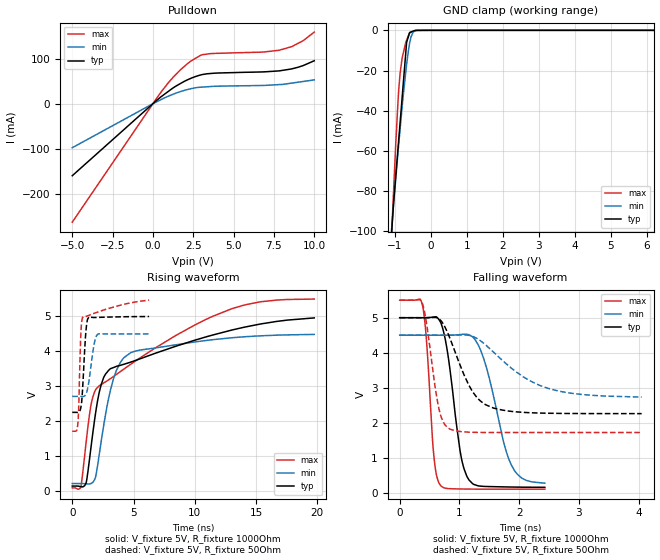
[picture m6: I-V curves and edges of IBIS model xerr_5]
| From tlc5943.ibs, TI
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|   xerr_5 Model
[Model]   xerr_5
Model_type   Open_drain
Polarity   Inverting
Vmeas = 2.5
Vref = 5.0
Cref = 15pF
Rref = 1000
|   typ   min   max
|   (nom PVT)   (Fast PVT)   (slow PVT)
C_comp   1.152e-12   1.144e-12   1.154e-12
|ON state : BUFFER OUTPUT TURNED LOW
|C_comp   2.072e-12   1.804e-12   2.153e-12
|OFF state: BUFFER IN HIGH IMPEDANCE
|C_comp   1.152e-12   1.144e-12   1.154e-12
| Where nom  PVT is Nominal Process,  5V,  65C
|   Fast PVT is Strong Process,   5.5V,  -40C
|   Slow PVT is Weak Process,   4.5V,  125C
[Voltage Range]   5   4.5   5.5
|Ambient Temperature   25   85   -40
|Junction Temperature
[Temperature Range]   65   125   -40
[Pullup Reference]   5   4.5   5.5
[Pulldown Reference]   0   0   0
[Power Clamp Reference]   5   4.5   5.5
[GND Clamp Reference]   0   0   0
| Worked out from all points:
|   slope of the pulldown table from 0 to 0.75 V, typ, clamps not added: 34.3 ohm
|   GND clamp passes 1 mA (typ) near -0.58 V on its own axis
|   falling waveform, V_fixture 5V, R_fixture 1000Ohm: 20-80 % time 220ps typ, 357ps min, 120ps max; typ from 5 V to 0.155 V
|   rising waveform, V_fixture 5V, R_fixture 1000Ohm: 20-80 % time 5.71ns typ, 1.64ns min, 7.21ns max; typ from 0.153 V to 4.96 V
|   rising waveform, V_fixture 5V, R_fixture 50Ohm: 20-80 % time 264ps typ, 426ps min, 205ps max; typ from 2.26 V to 5 V
|   falling waveform, V_fixture 5V, R_fixture 50Ohm: 20-80 % time 422ps typ, 830ps min, 190ps max; typ from 5 V to 2.26 V
[Pulldown]
|   Voltage   I(typ)   I(min)   I(max)
-5V       -159.5mA   -97.5mA    -262.4mA
561mV     16.88mA    10.08mA    28.48mA
1.282V    35.65mA    21.46mA    59.67mA
2.139V    52.88mA    31.32mA    88.62mA
2.376V    56.58mA    33.39mA    94.99mA
3.08V     64.69mA    36.82mA    108.6mA
4.02V     67.96mA    38.74mA    111.6mA
6.88V     70.5mA     40.46mA    114.5mA
7.827V    72.69mA    42.31mA    118.4mA
8.602V    77.1mA     45.59mA    126.4mA
9.312V    84.41mA    49.23mA    139.5mA
10V       95.12mA    52.76mA    158.6mA
[GND Clamp]
|   Voltage   I(typ)   I(min)   I(max)
-5V       -1.388A    -1.121A    -1.957A
-1.073V   -96.77mA   -95.46mA   -95.79mA
-1.035V   -86.47mA   -86.99mA   -81mA
-973.5mV  -72.9mA    -74.09mA   -56.9mA
-907.5mV  -58.35mA   -60.28mA   -34.67mA
-852.5mV  -46.21mA   -49.37mA   -21.54mA
-792mV    -32.87mA   -37.6mA    -13.6mA
-670mV    -5.959mA   -16.9mA    -4.924mA
-585mV    -1.038mA   -6.236mA   -1.293mA
-549mV    -794.9uA   -3.318mA   -1.048mA
-435mV    -26.55uA   -370.6uA   -270.9uA
10V       0A         0A         0A
[POWER Clamp]
|   Voltage   I(typ)   I(min)   I(max)
-5V       0A         0A         0A
10V       0A         0A         0A
[Ramp]
R_load = 1000
|   typ   min   max
dV/dt_r   2.90821/5.97792e-09   2.56519/1.64474e-09   3.23936/7.21532e-09
dV/dt_f   2.90801/2.18946e-10   2.56315/3.6109e-10   3.23918/1.19704e-10
[Falling Waveform]
V_fixture = 5V
V_fixture_min = 4.5V
V_fixture_max = 5.5V
R_fixture = 1000Ohm
|   Time   V(typ)   V(min)   V(max)
0s        5V         4.5V       5.5V
380ps     4.999V     4.5V       5.373V
450ps     5V         4.5V       4.325V
570ps     5.019V     4.5V       1.09V
690ps     4.853V     4.499V     196.3mV
1.03ns    1.017V     4.521V     107mV
1.16ns    364.8mV    4.513V     104mV
1.41ns    180.2mV    3.814V     101.9mV
1.87ns    162.4mV    788.8mV    101.5mV
2.43ns    155.2mV    271.8mV    101.4mV
[Rising Waveform]
V_fixture = 5V
V_fixture_min = 4.5V
V_fixture_max = 5.5V
R_fixture = 1000Ohm
|   Time   V(typ)   V(min)   V(max)
0s        152.9mV    224.5mV    101.1mV
715ps     132.7mV    224.9mV    155.9mV
1.12ns    234.5mV    216.9mV    1.366V
1.51ns    1.207V     223.3mV    2.431V
1.87ns    2.157V     378.1mV    2.882V
2.56ns    3.251V     1.877V     3.098V
3.355ns   3.537V     3.206V     3.282V
4.78ns    3.696V     3.968V     3.635V
12.99ns   4.608V     4.39V      5.216V
19.75ns   4.958V     4.486V     5.497V
[Rising Waveform]
V_fixture = 5V
V_fixture_min = 4.5V
V_fixture_max = 5.5V
R_fixture = 50Ohm
|   Time   V(typ)   V(min)   V(max)
0s        2.259V     2.716V     1.72V
460ps     2.257V     2.716V     1.942V
530ps     2.262V     2.716V     2.444V
700ps     2.394V     2.714V     4.475V
840ps     2.902V     2.711V     4.97V
1.11ns    4.552V     2.776V     4.999V
1.35ns    4.98V      3.122V     5.03V
1.78ns    4.969V     4.198V     5.088V
2.08ns    4.972V     4.494V     5.126V
6.27ns    4.997V     4.5V       5.466V
[Falling Waveform]
V_fixture = 5V
V_fixture_min = 4.5V
V_fixture_max = 5.5V
R_fixture = 50Ohm
|   Time   V(typ)   V(min)   V(max)
0s        5V         4.5V       5.5V
380ps     5V         4.5V       5.408V
450ps     5V         4.5V       4.84V
660ps     4.963V     4.5V       2.379V
840ps     4.418V     4.501V     1.82V
1.21ns    2.917V     4.473V     1.727V
1.56ns    2.425V     4.035V     1.721V
2.08ns    2.294V     3.299V     1.72V
2.51ns    2.27V      2.968V     1.72V
4.05ns    2.26V      2.732V     1.72V
